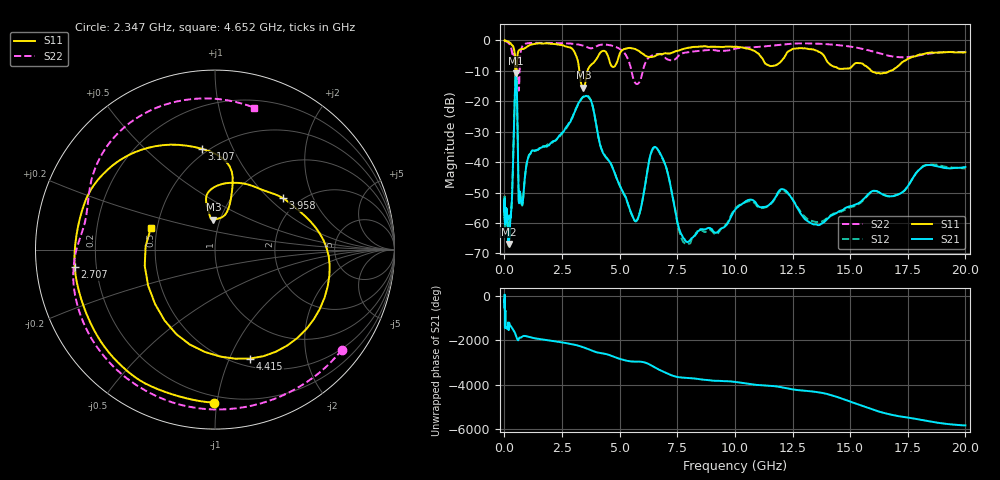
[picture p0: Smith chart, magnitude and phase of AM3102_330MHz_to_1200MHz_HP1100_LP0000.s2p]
! Date/Time: Tue, Sep 11, 2018 5:20 PM
! Network Analyzer: Agilent Technologies E8362B Rev: A.07.50.63
! Sweep from 0.010 to 20.000 GHz, 1601 Points, Sweep Type: LOG
! Power Supply: 4.949 V, 0.001 A
# Hz S DB R 50
!freq MagS11 AngS11 MagS21 AngS21 MagS12 AngS12 MagS22 AngS22
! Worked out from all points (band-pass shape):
!   1601 points, 10 MHz to 20 GHz, reference 50 ohm
!   highest |S21| = -10.79 dB at 503.6 MHz (marker M1); lowest = -66.9 dB at 188.4 MHz (marker M2)
!   |S21| within 3 dB of the highest: 471 MHz to 532.5 MHz (61.58 MHz wide, 12.3 % of centre)
!   lowest |S11| = -15.5 dB at 3.432 GHz (marker M3), VSWR 1.40, Z = 46.4 + j16 ohm
!   |S11| at or under -10 dB: 471.9 MHz to 528.1 MHz (56.2 MHz wide, 11.2 % of centre); 3.251 GHz to 3.606 GHz (354.6 MHz wide, 10.3 % of centre); 15.91 GHz to 16.76 GHz (842.6 MHz wide, 5.16 % of centre)
!   |S22| runs from -16.5 to -0.1 dB; largest |S21 - S12| = 0.0049
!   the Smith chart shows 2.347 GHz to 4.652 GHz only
!   S11 on the Smith chart (normalised r, x): 2.347 GHz: 0.16, -0.98; 2.707 GHz: 0.12, -0.06; 3.107 GHz: 0.46, +0.77; 3.958 GHz: 1.65, +1.22; 4.415 GHz: 0.58, -1.19; 4.652 GHz: 0.46, +0.13
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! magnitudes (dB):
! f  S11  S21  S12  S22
! 10 MHz  0.0  -53.3  -51.7  -0.1
! 35.55 MHz  -0.1  -57.7  -61.1  -0.2
! 126.4 MHz  -0.3  -58.8  -58.4  -0.6
! 188.4 MHz  -0.5  -66.9  -67.2  -1.0
! 320.7 MHz  -1.5  -53.2  -53.8  -3.5
! 447.2 MHz  -4.5  -19.1  -19.1  -4.4
! 503.6 MHz  -13.9  -10.8  -10.8  -10.0
! 632.6 MHz  -3.3  -53.4  -53.5  -16.2
! 757.7 MHz  -2.8  -53.9  -54.1  -2.3
! 1.59 GHz  -1.0  -35.3  -35.2  -0.8
! 2.347 GHz  -1.4  -31.7  -32.1  -0.9
! 2.707 GHz  -2.1  -28.2  -28.6  -1.0
! 3.107 GHz  -4.9  -22.3  -22.5  -1.2
! 3.432 GHz  -15.5  -18.5  -18.6  -1.8
! 3.958 GHz  -6.5  -26.7  -26.5  -2.1
! 4.415 GHz  -3.9  -38.5  -38.4  -1.4
! 4.652 GHz  -8.5  -41.1  -41.1  -1.7
! 5.652 GHz  -2.8  -59.2  -59.2  -13.7
! 6.549 GHz  -5.1  -35.0  -35.3  -4.6
! 7.958 GHz  -2.5  -66.3  -67.1  -3.9
! 13.68 GHz  -3.9  -60.7  -59.7  -1.1
! 20 GHz  -3.9  -41.6  -42.1  -3.8
